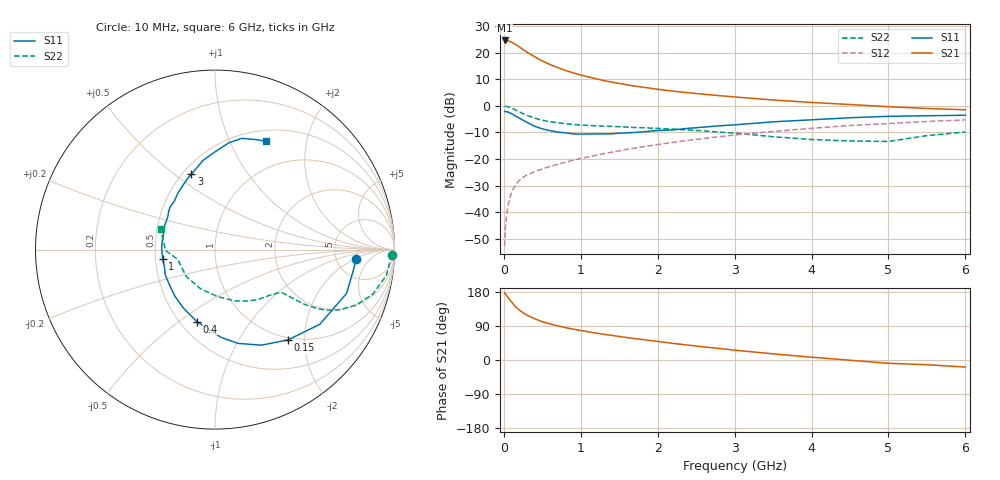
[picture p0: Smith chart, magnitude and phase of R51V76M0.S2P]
! SIEMENS Small Signal Semiconductors
! BFR183
! Si NPN RF Bipolar Junction Transistor in SOT23
! VCE = 1.75 V  IC = 6 mA
! Common Emitter S-Parameters:  May  1996
# GHz  S  MA  R  50
!  f  S11  S21  S12  S22
! GHz  MAG  ANG  MAG  ANG  MAG  ANG  MAG  ANG
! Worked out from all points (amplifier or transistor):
!   36 points, 10 MHz to 6 GHz, reference 50 ohm
!   highest |S21| = 24.6 dB at 10 MHz (marker M1)
!   |S21| within 3 dB of that: start of sweep to 228.8 MHz
!   unconditionally stable (mu >= 1): 928.5 MHz to 2.623 GHz
!   at 250 MHz: K = 0.47, MSG = 24.0 dB, |S12| = -26.9 dB
!   at 1.4 GHz: K = 1.07, MAG = 11.6 dB, |S12| = -17.4 dB
!   at 6 GHz: K = 0.90, MSG = 1.9 dB, |S12| = -5.3 dB
!   S11 on the Smith chart (normalised r, x): 10 MHz: 7.75, -2.18; 150 MHz: 0.96, -1.66; 400 MHz: 0.60, -0.58; 1 GHz: 0.55, -0.06; 3 GHz: 0.55, +0.58; 6 GHz: 0.63, +1.38
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0.01  0.7866 -3.9  17.03 177.3  0.0023 90.0  0.988 -1.7
0.02  0.7813 -7.4  17 174.2  0.0051 83.8  0.9785 -3.4
0.05  0.7728 -18.4  16.94 165.9  0.0126 81.1  0.9662 -8.5
0.1  0.7169 -35.5  15.81 153.1  0.0236 73.4  0.9126 -15.9
0.15  0.6472 -51.0  14.36 141.1  0.0327 66.6  0.8438 -21.5
0.2  0.5924 -64.0  12.94 132.1  0.0396 62.5  0.7745 -25.6
0.25  0.5385 -76.1  11.45 124.6  0.0454 59.8  0.7142 -28.2
0.3  0.4901 -86.1  10.26 118.3  0.0504 57.9  0.6663 -29.8
0.4  0.4139 -104.1  8.423 108.9  0.0581 56.9  0.5883 -31.4
0.5  0.3705 -118.4  6.989 101.1  0.0651 56.4  0.5366 -31.9
0.6  0.3421 -130.9  6.007 95.3  0.0727 56.9  0.5056 -32.1
0.8  0.3113 -152.7  4.66 85.5  0.0869 57.9  0.4631 -32.5
1  0.2953 -169.8  3.815 77.8  0.1025 59.3  0.4381 -33.2
1.1  0.2963 -177.4  3.505 74.4  0.1102 59.5  0.4296 -34.2
1.3  0.2979 169.8  3.001 68.0  0.1264 59.6  0.4165 -35.9
1.6  0.3112 154.0  2.491 59.2  0.1518 59.2  0.3987 -39.6
2.2  0.3538 129.6  1.895 43.9  0.2062 56.2  0.3666 -49.3
3  0.4411 107.3  1.475 26.0  0.284 48.9  0.3079 -68.5
3.5  0.5019 97.6  1.293 16.2  0.3311 43.0  0.2634 -86.0
4.5  0.5993 82.7  1.062 -0.6  0.4286 30.7  0.2192 -137.1
5.5  0.6526 70.1  0.896 -12.4  0.5091 18.4  0.2761 -178.9
6  0.6677 64.7  0.844 -18.6  0.5457 10.3  0.3228 159.4
